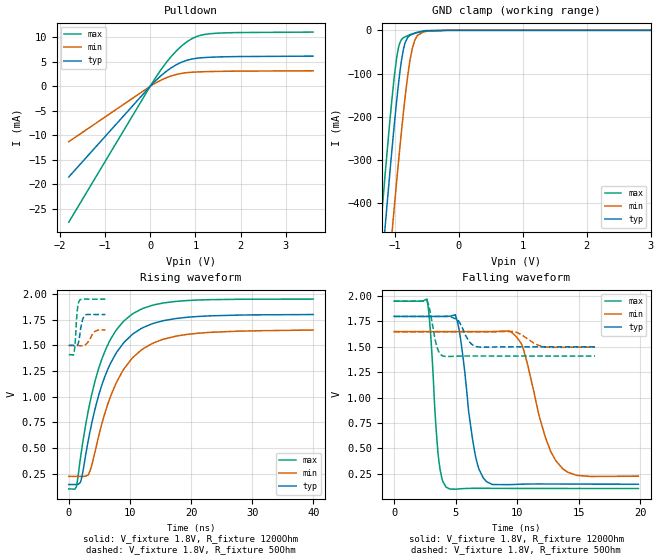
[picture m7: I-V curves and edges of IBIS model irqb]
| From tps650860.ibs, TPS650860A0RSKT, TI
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|   irqb Model
[Model]   irqb
Model_type   Open_drain
Polarity   Non-Inverting
Vmeas = 0.9
Vref = 1.8
Cref = 2pF
Rref = 1200
|   typ   min   max
|   (nom PVT)   (fast PVT)   (slow PVT)
C_comp   1.956e-12   1.893e-12   2.046e-12
| Where nom  PVT is Nominal Process, 1.8V, 27C
|   Fast PVT is Strong Process,  1.95V, -40C
|   Slow PVT is Weak Process,   1.65V, 125C
[Voltage Range]   1.8   1.65   1.95
|Junction Temperature
[Temperature Range]   27   125   -40
[Pullup Reference]   1.8   1.65   1.95
[Pulldown Reference]   0   0   0
[Power Clamp Reference]   1.8   1.65   1.95
[GND Clamp Reference]   0   0   0
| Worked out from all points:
|   slope of the pulldown table from 0 to 0.27 V, typ, clamps not added: 112 ohm
|   falling waveform, V_fixture 1.8V, R_fixture 1200Ohm: 20-80 % time 1.01ns typ, 1.84ns min, 561ps max; typ from 1.8 V to 0.146 V
|   rising waveform, V_fixture 1.8V, R_fixture 1200Ohm: 20-80 % time 5.39ns typ, 5.75ns min, 4.98ns max; typ from 0.146 V to 1.8 V
|   falling waveform, V_fixture 1.8V, R_fixture 50Ohm: 20-80 % time 746ps typ, 1.14ns min, 505ps max; typ from 1.8 V to 1.5 V
|   rising waveform, V_fixture 1.8V, R_fixture 50Ohm: 20-80 % time 514ps typ, 875ps min, 365ps max; typ from 1.5 V to 1.8 V
[Pulldown]
|   Voltage   I(typ)   I(min)   I(max)
-1.8V     -18.55mA   -11.33mA   -27.78mA
115.2mV   1.103mA    646.7uA    1.704mA
252mV     2.272mA    1.309mA    3.566mA
467.8mV   3.789mA    2.114mA    6.119mA
637.1mV   4.681mA    2.537mA    7.761mA
790.2mV   5.253mA    2.768mA    8.95mA
1.025V    5.724mA    2.927mA    10.16mA
1.33V     5.941mA    3.016mA    10.75mA
1.98V     6.08mA     3.099mA    10.99mA
3.6V      6.165mA    3.169mA    11.08mA
[GND Clamp]
|   Voltage   I(typ)   I(min)   I(max)
-1.8V     -1.644A    -1.827A    -1.538A
-1.203V   -549.4mA   -745.5mA   -428.8mA
-1.168V   -488mA     -684.2mA   -367.2mA
-1.122V   -408.2mA   -604.2mA   -287.5mA
-1.055V   -296.2mA   -490.4mA   -178.3mA
-1.015V   -232.1mA   -423.6mA   -119.2mA
-943.2mV  -128.1mA   -309.1mA   -42.29mA
-840.6mV  -30.72mA   -159.8mA   -15.18mA
-721.8mV  -8.712mA   -40.6mA    -8.088mA
-643.3mV  -5.218mA   -11.77mA   -4.432mA
-548.1mV  -2.161mA   -3.772mA   -1.292mA
3.6V      0A         0A         0A
[POWER Clamp]
|   Voltage   I(typ)   I(min)   I(max)
-1.8V     0A         0A         0A
0V        0A         0A         0A
3.6V      0A         0A         0A
[Ramp]
R_load = 1200
|   typ   min   max
dV/dt_r   0.992389/5.36262e-09   0.854474/5.74389e-09   1.1078/4.95934e-09
dV/dt_f   0.992455/1.0041e-09   0.854839/1.81104e-09   1.10781/5.58639e-10
[Falling Waveform]
V_fixture = 1.8V
V_fixture_min = 1.65V
V_fixture_max = 1.95V
R_fixture = 1200Ohm
|   Time   V(typ)   V(min)   V(max)
0s        1.8V       1.65V      1.95V
2.675ns   1.8V       1.65V      1.971V
3.58ns    1.8V       1.65V      442.9mV
4.23ns    1.8V       1.65V      117.2mV
5.165ns   1.74V      1.65V      98.48mV
6.52ns    484mV      1.65V      105.8mV
7.49ns    173.2mV    1.65V      105.7mV
10.35ns   146.5mV    1.531V     104.4mV
13.7ns    147.8mV    298.2mV    104mV
19.85ns   145.9mV    225.2mV    103.7mV
[Rising Waveform]
V_fixture = 1.8V
V_fixture_min = 1.65V
V_fixture_max = 1.95V
R_fixture = 1200Ohm
|   Time   V(typ)   V(min)   V(max)
0s        145.9mV    225mV      103.7mV
1.255ns   145.7mV    225.1mV    124.7mV
1.945ns   173.7mV    224.7mV    416.1mV
3.47ns    660.6mV    277.2mV    945mV
5.405ns   1.113V     736.8mV    1.365V
7.69ns    1.419V     1.126V     1.642V
10.28ns   1.6V       1.368V     1.8V
13.54ns   1.708V     1.514V     1.888V
17.52ns   1.761V     1.589V     1.928V
39.95ns   1.8V       1.649V     1.95V
[Falling Waveform]
V_fixture = 1.8V
V_fixture_min = 1.65V
V_fixture_max = 1.95V
R_fixture = 50Ohm
|   Time   V(typ)   V(min)   V(max)
0s        1.8V       1.65V      1.95V
2.675ns   1.8V       1.65V      1.958V
3.48ns    1.8V       1.65V      1.502V
3.96ns    1.8V       1.65V      1.41V
5.225ns   1.759V     1.65V      1.409V
6.12ns    1.55V      1.65V      1.41V
6.77ns    1.5V       1.65V      1.41V
9.71ns    1.5V       1.652V     1.41V
12.32ns   1.5V       1.499V     1.409V
16.33ns   1.5V       1.498V     1.409V
[Rising Waveform]
V_fixture = 1.8V
V_fixture_min = 1.65V
V_fixture_max = 1.95V
R_fixture = 50Ohm
|   Time   V(typ)   V(min)   V(max)
0s        1.5V       1.498V     1.409V
830ps     1.499V     1.498V     1.42V
1.03ns    1.498V     1.498V     1.511V
1.255ns   1.499V     1.498V     1.74V
1.38ns    1.501V     1.497V     1.829V
1.74ns    1.574V     1.497V     1.935V
2.22ns    1.742V     1.496V     1.95V
2.595ns   1.789V     1.501V     1.95V
4.285ns   1.8V       1.636V     1.95V
5.998ns   1.8V       1.65V      1.95V
